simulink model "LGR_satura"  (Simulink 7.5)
settings: Solver=ode45  StartTime=0.0  StopTime=50  RelTol=1e-8
libraries: simulink x1

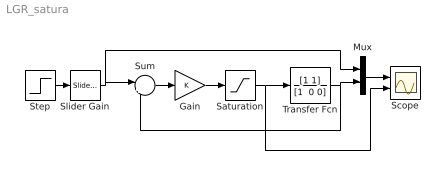
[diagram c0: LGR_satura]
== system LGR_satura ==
  Gain : Gain  ParameterDataType=fixdt(1, 16)  ParameterScaling=2^0  OutDataType=fixdt(1, 16)  OutScaling=2^0
  Mux : Mux  Inputs=2
  Saturation : Saturate  UpperLimit=.1  LowerLimit=-.1  OutDataType=fixdt(1, 16)  OutScaling=2^0
  Scope : Scope  NumInputPorts=2
  Slider Gain : simulink/Math Operations/Slider Gain  SystemSampleTime=-1  low=0  gain=0.1  high=100
  Step : Step  Time=0  SampleTime=0
  Sum : Sum  Inputs=|+-  OutDataType=fixdt(1, 16)  OutScaling=2^0
  Transfer Fcn : TransferFcn  Numerator=[1 1]  Denominator="[1  0 0]"
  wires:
  Step/1 -> Slider Gain/1
  Slider Gain/1 -> Sum/1, Mux/1
  Sum/1 -> Gain/1
  Gain/1 -> Saturation/1
  Saturation/1 -> Transfer Fcn/1, Scope/2
  Mux/1 -> Scope/1
  Transfer Fcn/1 -> Mux/2, Sum/2
